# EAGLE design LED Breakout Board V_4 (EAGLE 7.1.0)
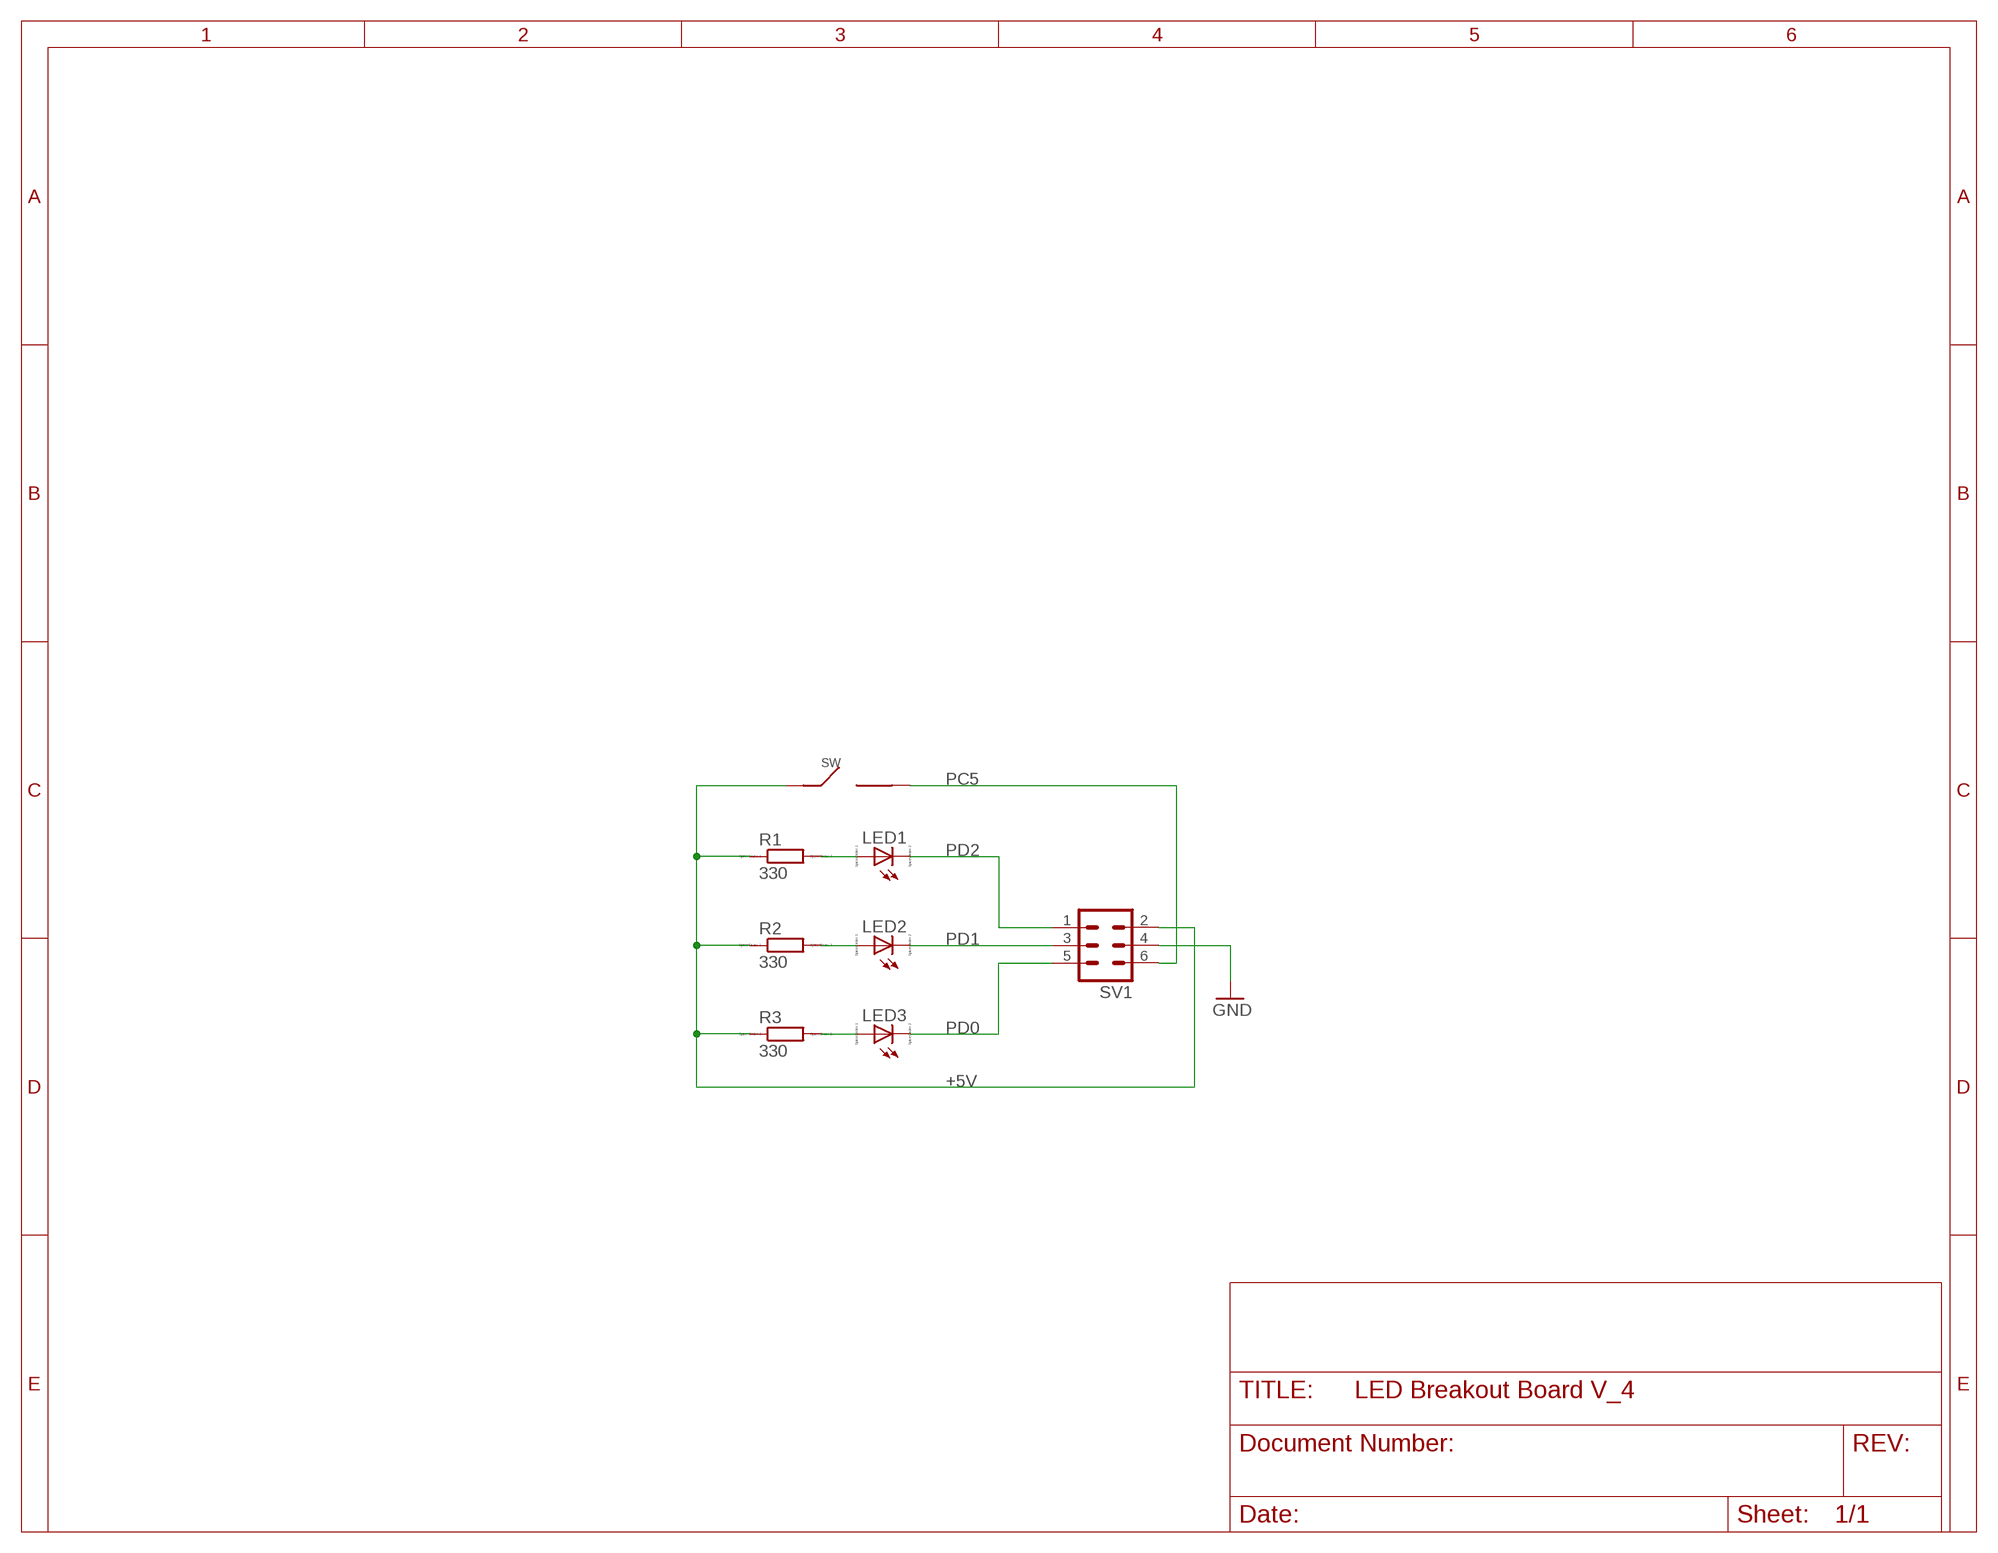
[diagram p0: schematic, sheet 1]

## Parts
LED1  LED_ELD260  [LED_LD260]
LED2  LED_ELD260  [LED_LD260]
LED3  LED_ELD260  [LED_LD260]
R1  330  R-EU_R0805  [R0805]
R2  330  R-EU_R0805  [R0805]
R3  330  R-EU_R0805  [R0805]
SV1  MA03-2  [MA03-2]
SW  PUSHBUTTON  [PUSHBUTTON]

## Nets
+5V: R1.1 R2.1 R3.1 SV1.2 SW.IN
GND: SV1.4
N$1: LED3.A R3.2
N$2: LED2.A R2.2
N$3: LED1.A R1.2
PC5: SV1.6 SW.OUT
PD0: LED3.K(C) SV1.5
PD1: LED2.K(C) SV1.3
PD2: LED1.K(C) SV1.1

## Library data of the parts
LED1-LED3 = eagle-ltspice:LED_E: LED; SPICEMODEL: NONE; SPICEPREFIX: D; SPICETYPE: diode
R1-R3 = resistor:R-EU_: RESISTOR, European symbol; SPICEPREFIX: R
SV1 = con-lstb:MA03-2: PIN HEADER; OC_FARNELL: unknown; OC_NEWARK: unknown
SW = pushbutton:PUSHBUTTON

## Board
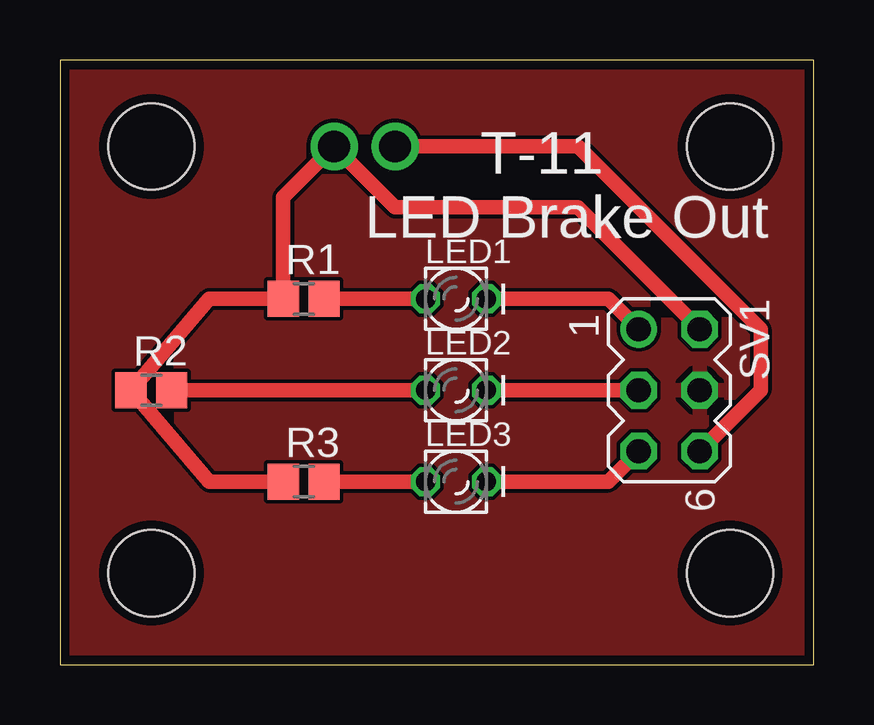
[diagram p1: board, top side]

Size 31.42 x 25.19 mm. Coordinates in mm from the lower left corner, seen from the top.
Outline: 0,0 31.42,0 31.42,25.19 0,25.19 0,0
Copper layers (1*16): Top 0.0356mm / dielectric 1.5011mm / Bottom 0.0356mm
Design rules "OHS-Park": minimum track width 6mil, minimum drill 13mil, track to track 6mil, track to pad 6mil, pad to pad 6mil, via to via 6mil, smd to smd 6mil, copper to edge 15mil, drill to drill 6mil, minimum pad ring 7mil, minimum via ring 7mil, stop-mask expansion 3mil, vias tented up to drill 0mil, thermal gap 10mil
Holes 3.6 mm at 3.81,21.59 27.94,21.59 27.94,3.81 3.81,3.81

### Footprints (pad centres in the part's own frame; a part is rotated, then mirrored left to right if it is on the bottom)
LED_LD260 = drill 0.813 octagon: A -1.27,0; K 1.27,0
R0805 = smd 1.3 x 1.5: 1 -0.85,0; 2 0.85,0
MA03-2 = drill 1.016: 1 -2.54,-1.27 | drill 1.016 octagon: 2 -2.54,1.27; 3 0,-1.27; 4 0,1.27; 5 2.54,-1.27; 6 2.54,1.27
PUSHBUTTON = drill 1.321: IN -1.27,0; OUT 1.27,0

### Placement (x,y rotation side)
LED1  16.51,15.24 0 top
LED2  16.51,11.43 0 top
LED3  16.51,7.62 0 top
R1  10.16,15.24 0 top
R2  3.81,11.43 0 top
R3  10.16,7.62 0 top
SV1  25.4,11.43 270 top
SW  12.7,21.59 0 top

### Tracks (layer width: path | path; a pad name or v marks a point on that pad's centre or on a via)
+5V
  Top 0.61: R3.1 6.22,7.62 R2.1 6.22,15.24 R1.1 9.31,19.47 SW.IN 13.97,19.05 21.59,19.05 SV1.2
GND
  pour Top: 0,25.53 30.98,25.73 30.98,0.11 0,-0.09
N$1
  Top 0.61: R3.2 LED3.A
N$2
  Top 0.61: R2.2 LED2.A
N$3
  Top 0.61: R1.2 LED1.A
PC5
  Top 0.61: SW.OUT 21.59,21.59 29.21,13.97 29.21,11.43 SV1.6
PD0
  Top 0.61: LED3.K 22.86,7.62 SV1.5
PD1
  Top 0.61: LED2.K SV1.3
PD2
  Top 0.61: LED1.K 22.86,15.24 SV1.1

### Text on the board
tNames: T-11 / LED Brake Out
